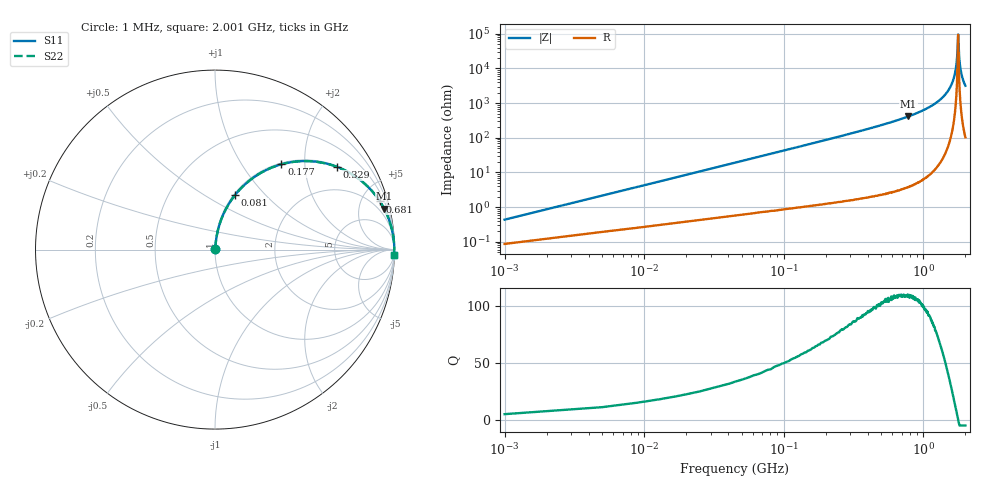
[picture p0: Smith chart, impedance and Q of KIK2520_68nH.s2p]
!version-2
!date-01.2022
!Series
# MHz S RI R 50
!Freq ReS11 ImS11 ReS21 ImS21 ReS12 ImS12 ReS22 ImS22
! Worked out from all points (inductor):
!   501 points, 1 MHz to 2.001 GHz, reference 50 ohm
!   read as one part in series: L = 68 nH near 9 MHz
!   highest Q = 109 at 781 MHz (marker M1), where L = 84.3 nH
!   self-resonance near 1.773 GHz
!   S11 on the Smith chart (normalised r, x): 1 MHz: 1.00, +0.01; 81 MHz: 1.02, +0.69; 177 MHz: 1.02, +1.53; 329 MHz: 1.03, +2.91; 681 MHz: 1.06, +6.82; 2.001 GHz: 3, -63
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1  0.000873 0.00426  0.9991 -0.00426  0.9991 -0.00426  0.000873 0.00426
13  0.00612 0.055  0.9939 -0.055  0.9939 -0.055  0.00612 0.055
25  0.0154 0.1047  0.9846 -0.1047  0.9846 -0.1047  0.0154 0.1047
49  0.0473 0.1984  0.9527 -0.1984  0.9527 -0.1984  0.0473 0.1984
81  0.1128 0.3053  0.8872 -0.3053  0.8872 -0.3053  0.1128 0.3053
177  0.3704 0.4754  0.6296 -0.4754  0.6296 -0.4754  0.3704 0.4754
329  0.6775 0.4617  0.3225 -0.4617  0.3225 -0.4617  0.6775 0.4617
337  0.6886 0.4575  0.3114 -0.4575  0.3114 -0.4575  0.6886 0.4575
669  0.9152 0.274  0.0848 -0.274  0.0848 -0.274  0.9152 0.274
681  0.9188 0.2686  0.0812 -0.2686  0.0812 -0.2686  0.9188 0.2686
781  0.9429 0.2274  0.057 -0.2274  0.057 -0.2274  0.9429 0.2274
1001  0.9737 0.155  0.0263 -0.155  0.0263 -0.155  0.9737 0.155
1337  0.9931 0.0752  0.00687 -0.0752  0.00687 -0.0752  0.9931 0.0752
1541  0.9975 0.0373  0.00247 -0.0373  0.00247 -0.0373  0.9975 0.0373
1669  0.9987 0.0163  0.0013 -0.0163  0.0013 -0.0163  0.9987 0.0163
1733  0.9989 0.00637  0.00106 -0.00637  0.00106 -0.00637  0.9989 0.00637
1769  0.999 0.000963  0.00102 -0.000963  0.00102 -0.000963  0.999 0.000963
1777  0.999 -0.000224  0.00102 0.000224  0.00102 0.000224  0.999 -0.000224
1809  0.999 -0.00492  0.00104 0.00492  0.00104 0.00492  0.999 -0.00492
1845  0.9989 -0.0101  0.00112 0.0101  0.00112 0.0101  0.9989 -0.0101
1909  0.9986 -0.0191  0.00138 0.0191  0.00138 0.0191  0.9986 -0.0191
2001  0.998 -0.0314  0.00201 0.0314  0.00201 0.0314  0.998 -0.0314
